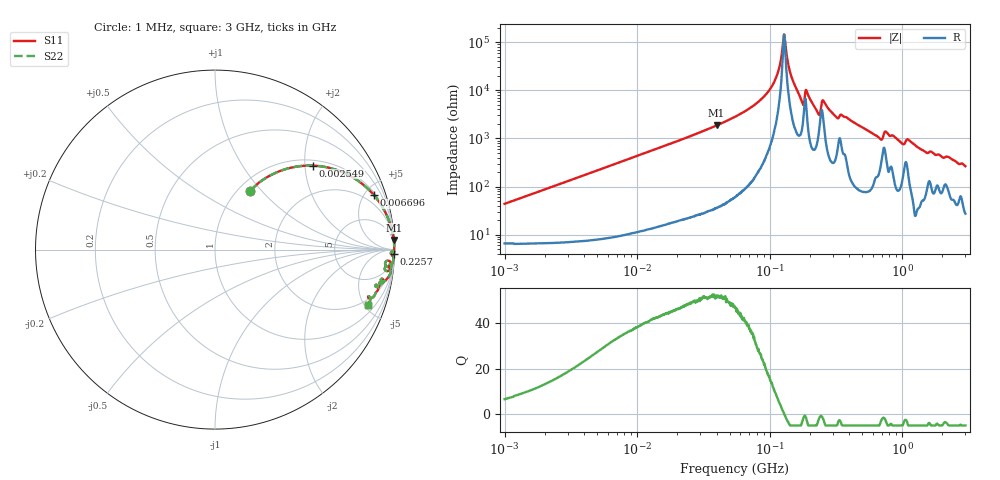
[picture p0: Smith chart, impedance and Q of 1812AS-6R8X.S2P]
!s-Parameter Generated by FASTRON Sdn. Bhd.
!FASTRON P/N : 1812AS-6R8X
!Keysight Technologies,E4991B,MY54100416,A.01.15
!Date created: Fri Oct 13 16:06:22 2023
!Version  : Rev00 Fri Oct 13 16:06:22 2023
!Data & Calibration Information:
!Freq	S11	S21	S12	S22
!PortZ  Port1:50+j0  Port2:50+j0
!When reading, reference impedance value at option line is always used.
! Remarks : This data is being provided solely for informational purposes.
# Hz S dB R 50
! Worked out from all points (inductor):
!   1601 points, 1 MHz to 3 GHz, reference 50 ohm
!   read as one part in series: L = 6.9 uH near 1.041 MHz
!   highest Q = 52.1 at 39.76 MHz (marker M1), where L = 7.44 uH
!   self-resonance near 128.2 MHz
!   S11 on the Smith chart (normalised r, x): 1 MHz: 1.13, +0.87; 2.549 MHz: 1.14, +2.21; 6.696 MHz: 1.18, +5.79; 225.7 MHz: 15, -76; 3 GHz: 1.55, -5.27
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1000000  -8.38 59.2  -1.22 -22.1  -1.22 -22.1  -8.38 59.2
2549110  -2.86 40.5  -3.73 -45.9  -3.73 -45.9  -2.86 40.5
3804036  -1.53 30.6  -5.87 -56.9  -5.87 -56.9  -1.53 30.6
6696013  -0.57 18.9  -9.81 -69.4  -9.81 -69.4  -0.57 18.9
1.447069e7  -0.14 9.0  -16.10 -79.6  -16.10 -79.6  -0.14 9.0
3.976269e7  -0.02 3.1  -25.41 -85.8  -25.41 -85.8  -0.02 3.1
5.477226e7  -0.01 2.0  -28.99 -86.7  -28.99 -86.7  -0.01 2.0
1.008535e8  -0.01 0.5  -40.55 -85.6  -40.55 -85.6  -0.01 0.5
1.148668e8  -0.01 0.3  -47.03 -81.5  -47.03 -81.5  -0.01 0.3
1.282345e8  -0.01 0.0  -63.20 -13.4  -63.20 -13.4  -0.01 0.0
1.453231e8  -0.01 -0.3  -46.04 80.0  -46.04 80.0  -0.01 -0.3
1.731398e8  -0.03 -0.9  -36.08 77.2  -36.08 77.2  -0.03 -0.9
1.923242e8  -0.03 -0.6  -39.02 73.8  -39.02 73.8  -0.03 -0.6
2.083556e8  -0.02 -1.0  -34.98 82.5  -34.98 82.5  -0.02 -1.0
2.257233e8  -0.04 -1.5  -31.75 77.9  -31.75 77.9  -0.04 -1.5
2.349428e8  -0.12 -1.7  -29.98 63.7  -29.98 63.7  -0.12 -1.7
2.570867e8  -0.05 -0.9  -35.29 71.5  -35.29 71.5  -0.05 -0.9
3.204059e8  -0.06 -2.1  -28.73 78.2  -28.73 78.2  -0.06 -2.1
3.576934e8  -0.06 -1.9  -29.34 78.3  -29.34 78.3  -0.06 -1.9
6.787043e8  -0.23 -5.5  -20.12 71.7  -20.12 71.7  -0.23 -5.5
7.925923e8  -0.16 -4.7  -21.54 75.2  -21.54 75.2  -0.16 -4.7
3e9  -0.86 -19.9  -9.33 64.2  -9.33 64.2  -0.86 -19.9
